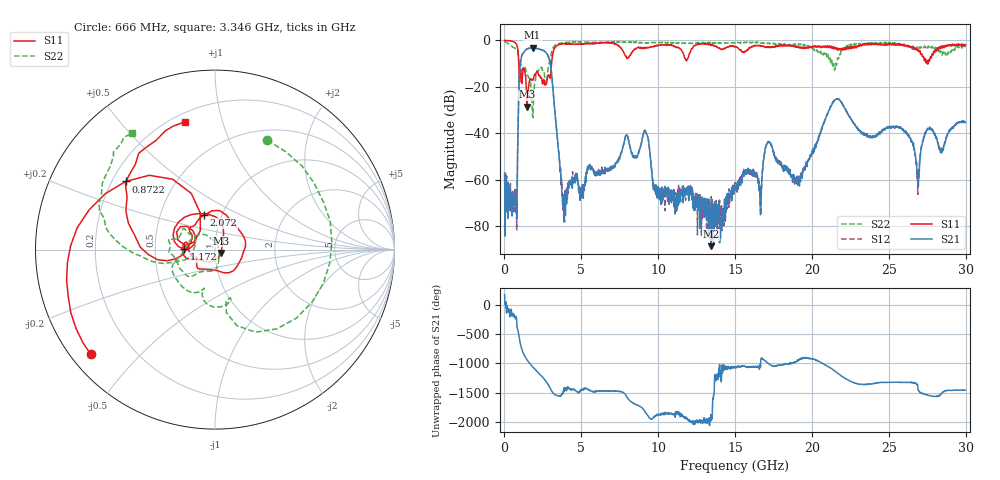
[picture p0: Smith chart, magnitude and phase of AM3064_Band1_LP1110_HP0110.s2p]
# Hz S DB R 50.0
!freq dBS11 angS11 dBS21 angS21 dBS12 angS12 dBS22 angS22
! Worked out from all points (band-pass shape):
!   1600 points, 10 MHz to 29.98 GHz, reference 50 ohm
!   highest |S21| = -3.21 dB at 1.828 GHz (marker M1); lowest = -88.7 dB at 13.43 GHz (marker M2)
!   |S21| within 3 dB of the highest: 1.154 GHz to 2.804 GHz (1.65 GHz wide, 83.4 % of centre)
!   lowest |S11| = -28.6 dB at 1.472 GHz (marker M3), VSWR 1.08, Z = 53.2 - j2.08 ohm
!   |S11| at or under -10 dB: 931.5 MHz to 3.062 GHz (2.131 GHz wide, 107 % of centre); 27.52151 GHz to 27.54909 GHz (27.58 MHz wide, 0.1 % of centre)
!   |S22| runs from -33.3 to -0.4 dB; largest |S21 - S12| = 0.0099
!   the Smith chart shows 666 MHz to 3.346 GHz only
!   S11 on the Smith chart (normalised r, x): 666 MHz: 0.06, -0.36; 872.2 MHz: 0.25, +0.32; 1.172 GHz: 0.71, +0.01; 2.072 GHz: 0.82, +0.33; 3.346 GHz: 0.25, +0.76
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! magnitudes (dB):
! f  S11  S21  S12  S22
! 10 MHz  0.0  -57.2  -57.6  -0.4
! 666 MHz  -0.9  -71.1  -64.4  -3.4
! 872.2 MHz  -4.1  -42.3  -42.2  -5.0
! 1.172 GHz  -15.3  -5.9  -5.9  -12.6
! 1.472 GHz  -28.6  -3.7  -3.7  -15.1
! 1.828 GHz  -16.9  -3.2  -3.2  -32.5
! 2.072 GHz  -13.9  -3.4  -3.5  -14.2
! 2.897 GHz  -14.9  -7.7  -7.6  -10.0
! 3.346 GHz  -2.7  -35.4  -35.4  -2.0
! 3.89 GHz  -1.4  -68.2  -71.1  -1.0
! 5.015 GHz  -1.5  -63.9  -65.1  -0.5
! 9.157 GHz  -3.5  -39.2  -38.9  -1.2
! 10 GHz  -2.2  -63.0  -67.0  -0.9
! 13.43 GHz  -1.9  -88.7  -71.6  -1.2
! 15 GHz  -2.7  -64.6  -61.3  -1.2
! 16.62 GHz  -2.1  -67.5  -67.2  -0.9
! 17.18 GHz  -2.7  -43.9  -43.5  -1.2
! 19.99 GHz  -3.1  -48.9  -48.7  -3.0
! 21.58 GHz  -3.6  -25.2  -25.2  -10.8
! 25 GHz  -1.4  -37.1  -37.6  -1.1
! 26.89 GHz  -4.0  -58.7  -66.4  -3.3
! 29.98 GHz  -1.9  -35.4  -35.1  -2.9
